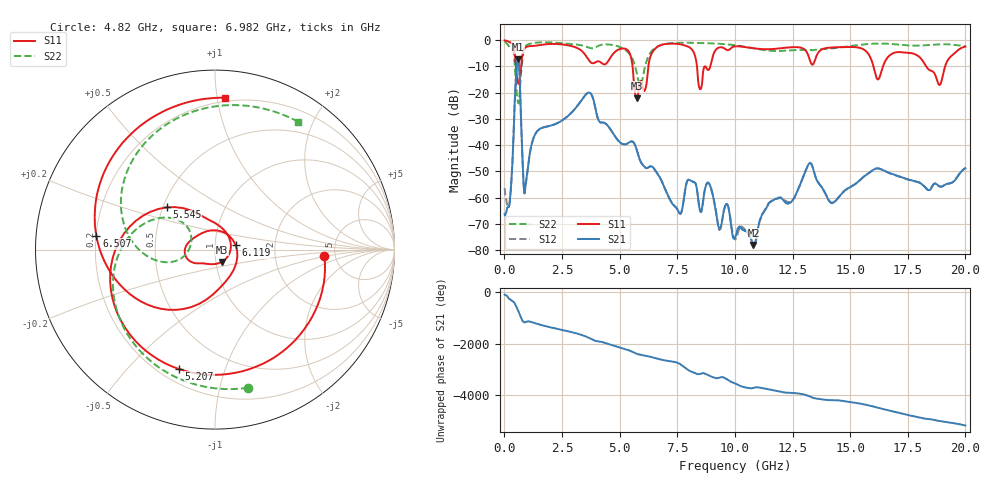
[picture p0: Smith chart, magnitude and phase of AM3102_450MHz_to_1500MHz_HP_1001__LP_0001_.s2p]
!Agilent Technologies,E8364B,MY43040894,A.07.50.67
!Agilent E8364B: A.07.50.67
!Date: Thursday, January 11, 2018 06:01:06
!Correction: S11(Full 2 Port(1,2))
!S21(Full 2 Port(1,2))
!S12(Full 2 Port(1,2))
!S22(Full 2 Port(1,2))
!S2P File: Measurements: S11, S21, S12, S22:
# Hz S  dB  R 50
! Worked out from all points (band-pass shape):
!   1601 points, 10 MHz to 20 GHz, reference 50 ohm
!   highest |S21| = -7.24 dB at 597.2 MHz (marker M1); lowest = -78.1 dB at 10.8 GHz (marker M2)
!   |S21| within 3 dB of the highest: 534.6 MHz to 642 MHz (107.4 MHz wide, 18.3 % of centre)
!   lowest |S11| = -22.1 dB at 5.745 GHz (marker M3), VSWR 1.17, Z = 53.4 - j7.35 ohm
!   |S11| at or under -10 dB: 5.56 GHz to 6.244 GHz (684 MHz wide, 11.6 % of centre); 16.01 GHz to 16.42 GHz (411.2 MHz wide, 2.54 % of centre); 18.3 GHz to 19.12 GHz (817 MHz wide, 4.37 % of centre)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
!   |S22| runs from -24.1 to -0.5 dB; largest |S21 - S12| = 0.0027
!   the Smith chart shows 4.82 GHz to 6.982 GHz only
!   S11 on the Smith chart (normalised r, x): 4.82 GHz: 4.08, -0.48; 5.207 GHz: 0.27, -0.71; 5.545 GHz: 0.52, +0.28; 6.119 GHz: 1.26, +0.06; 6.507 GHz: 0.20, +0.06; 6.982 GHz: 0.17, +1.05
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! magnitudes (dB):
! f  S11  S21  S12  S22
! 10 MHz  -0.1  -66.3  -56.4  -0.5
! 247.4 MHz  -0.8  -60.1  -60.1  -3.0
! 597.2 MHz  -16.4  -7.2  -7.2  -23.8
! 909.5 MHz  -2.8  -56.0  -56.1  -2.3
! 1.397 GHz  -2.0  -35.0  -35.0  -0.9
! 3.346 GHz  -4.0  -22.9  -22.9  -1.9
! 4.82 GHz  -4.3  -36.9  -36.9  -2.0
! 5.207 GHz  -3.2  -39.7  -39.7  -3.4
! 5.545 GHz  -8.9  -38.6  -38.6  -6.9
! 5.745 GHz  -22.1  -41.9  -41.9  -12.6
! 6.119 GHz  -18.6  -48.6  -48.6  -9.4
! 6.507 GHz  -3.5  -49.1  -49.2  -3.1
! 6.682 GHz  -2.3  -51.4  -51.4  -2.2
! 6.982 GHz  -1.4  -57.0  -56.8  -1.4
! 8.493 GHz  -18.7  -65.0  -65.2  -1.0
! 10.01 GHz  -2.3  -75.3  -75.9  -1.9
! 10.8 GHz  -3.0  -78.1  -78.1  -3.1
! 13.34 GHz  -9.2  -47.7  -47.6  -3.8
! 14.2 GHz  -2.7  -62.2  -61.9  -3.1
! 16.68 GHz  -6.1  -50.6  -50.6  -1.3
! 18.88 GHz  -17.1  -55.7  -55.7  -1.5
! 20 GHz  -2.4  -48.8  -48.9  -2.3
